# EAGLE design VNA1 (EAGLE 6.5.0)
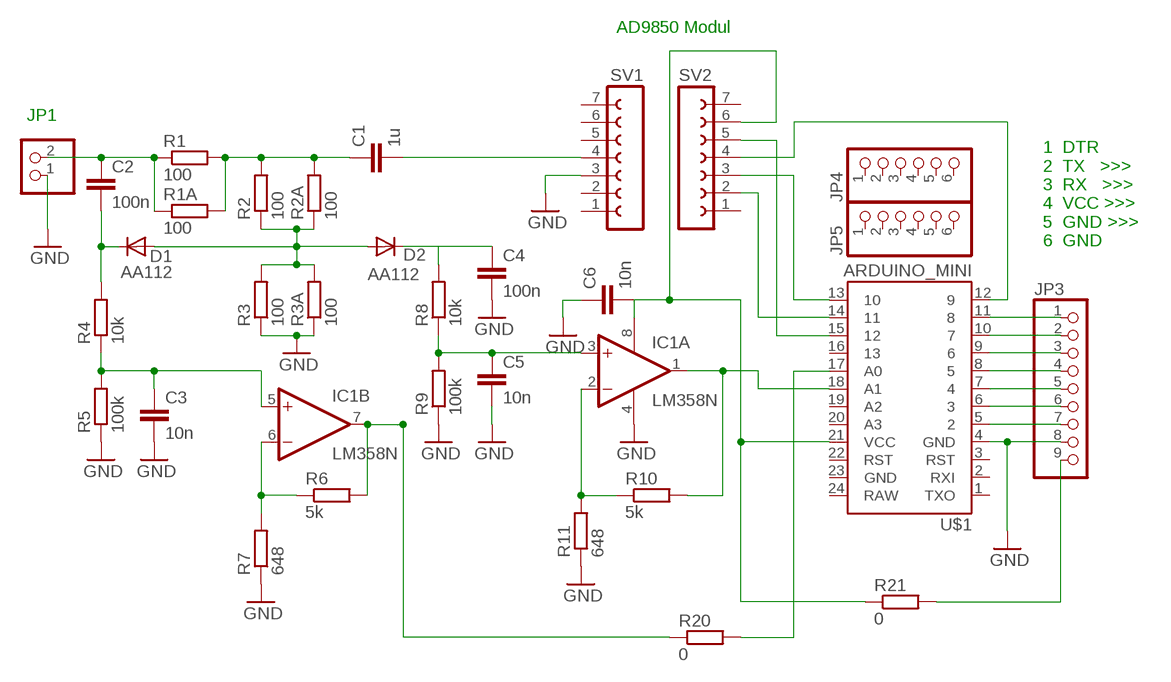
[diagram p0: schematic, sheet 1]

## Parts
C1  1u  C-EU025-040X050  [C025-040X050]
C2  100n  C-EU050-025X075  [C050-025X075]
C3  10n  C-EU050-025X075  [C050-025X075]
C4  100n  C-EU050-025X075  [C050-025X075]
C5  10n  C-EU050-025X075  [C050-025X075]
C6  10n  C-EU050-025X075  [C050-025X075]
D1  AA112  [DO07]
D2  AA112  [DO07]
IC1  LM358N  [DIL08]
JP1  PINHD-1X2  [1X02]
JP3  PINHD-1X9  [1X09]
JP4  PINHD-1X6  [1X06]
JP5  PINHD-1X6  [1X06]
R1  100  R-EU_0207/7  [0207/7]
R1A  100  R-EU_0207/7  [0207/7]
R2  100  R-EU_0207/7  [0207/7]
R2A  100  R-EU_0207/7  [0207/7]
R3  100  R-EU_0207/7  [0207/7]
R3A  100  R-EU_0207/7  [0207/7]
R4  10k  R-EU_0207/7  [0207/7]
R5  100k  R-EU_0207/7  [0207/7]
R6  5k  R-EU_0207/7  [0207/7]
R7  648  R-EU_0207/7  [0207/7]
R8  10k  R-EU_0207/7  [0207/7]
R9  100k  R-EU_0207/7  [0207/7]
R10  5k  R-EU_0207/7  [0207/7]
R11  648  R-EU_0207/7  [0207/7]
R20  0  R-EU_0207/7  [0207/7]
R21  0  R-EU_0207/7  [0207/7]
SV1  FE07-1  [FE07]
SV2  FE07-1  [FE07]
U$1  ARDUINO_MINI  [ARDUINO_MINI]

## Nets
GND: C3.2 C4.2 C5.2 C6.1 IC1.4(P:V-) JP1.1 JP3.8 R3.1 R3A.1 R5.1 R7.1 R9.1 R11.1 SV1.3 U$1.4(GND)
N$1: C3.1 IC1.5(B:+IN) R4.1 R5.2
N$2: C2.1 JP1.2 R1.1 R1A.1
N$3: C1.1 R1.2 R1A.2 R2.2 R2A.2
N$4: C2.2 D1.C R4.2
N$5: D1.A D2.A R2.1 R2A.1 R3.2 R3A.2
N$6: IC1.6(B:-IN) R6.1 R7.2
N$7: C4.1 D2.C R8.2
N$8: IC1.7(B:OUT) R6.2 R20.1
N$9: C5.1 IC1.3(A:+IN) R8.1 R9.2
N$10: IC1.2(A:-IN) R10.1 R11.2
N$12: C1.2 SV1.4
N$14: C6.2 IC1.8(P:V+) R21.1 SV2.6 U$1.21(VCC)
N$15: SV2.5 U$1.15
N$16: SV2.3 U$1.13
N$17: SV2.4 U$1.12
N$18: SV2.2 U$1.14
N$19: R20.2 U$1.17(A0)
N$20: JP3.9 R21.2
N$21: JP3.1 U$1.11
N$22: JP3.2 U$1.10
N$23: JP3.3 U$1.9
N$24: JP3.4 U$1.8
N$25: JP3.5 U$1.7
N$26: JP3.6 U$1.6
N$27: JP3.7 U$1.5
N$28: IC1.1(A:OUT) R10.2 U$1.18(A1)
Unconnected: JP4.1 JP4.2 JP4.3 JP4.4 JP4.5 JP4.6 JP5.1 JP5.2 JP5.3 JP5.4 JP5.5 JP5.6 SV1.1 SV1.2 SV1.5 SV1.6 SV1.7 SV2.1 SV2.7 U$1.1(TXO) U$1.2(RXI) U$1.3(RST) U$1.16 U$1.19(A2) U$1.20(A3) U$1.22(RST) U$1.23(GND) U$1.24(RAW)

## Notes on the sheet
- AD9850 Modul
- 1  DTR
  2  TX   >>>
  3  RX   >>>
  4  VCC >>>
  5  GND >>>
  6  GND

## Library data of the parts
C1-C6 = resistor:C-EU: CAPACITOR, European symbol
D1 D2 = diode:AA112: DIODE
IC1 = linear:LM358: OP AMP also LM158; LM258; LM2904 Source: http://cache.national.com/ds/LM/LM158.pdf
JP1 = pinhead:PINHD-1X2: PIN HEADER
JP3 = pinhead:PINHD-1X9: PIN HEADER
JP4 JP5 = pinhead:PINHD-1X6: PIN HEADER
R1 R1A R2 R2A R3 R3A R4-R11 R20 R21 = resistor:R-EU_: RESISTOR, European symbol
SV1 SV2 = con-lsta:FE07-1: FEMALE HEADER; OC_FARNELL: unknown; OC_NEWARK: unknown
U$1 = sparkfun_boards:ARDUINO_MINI: Arduino Pro Mini footprint

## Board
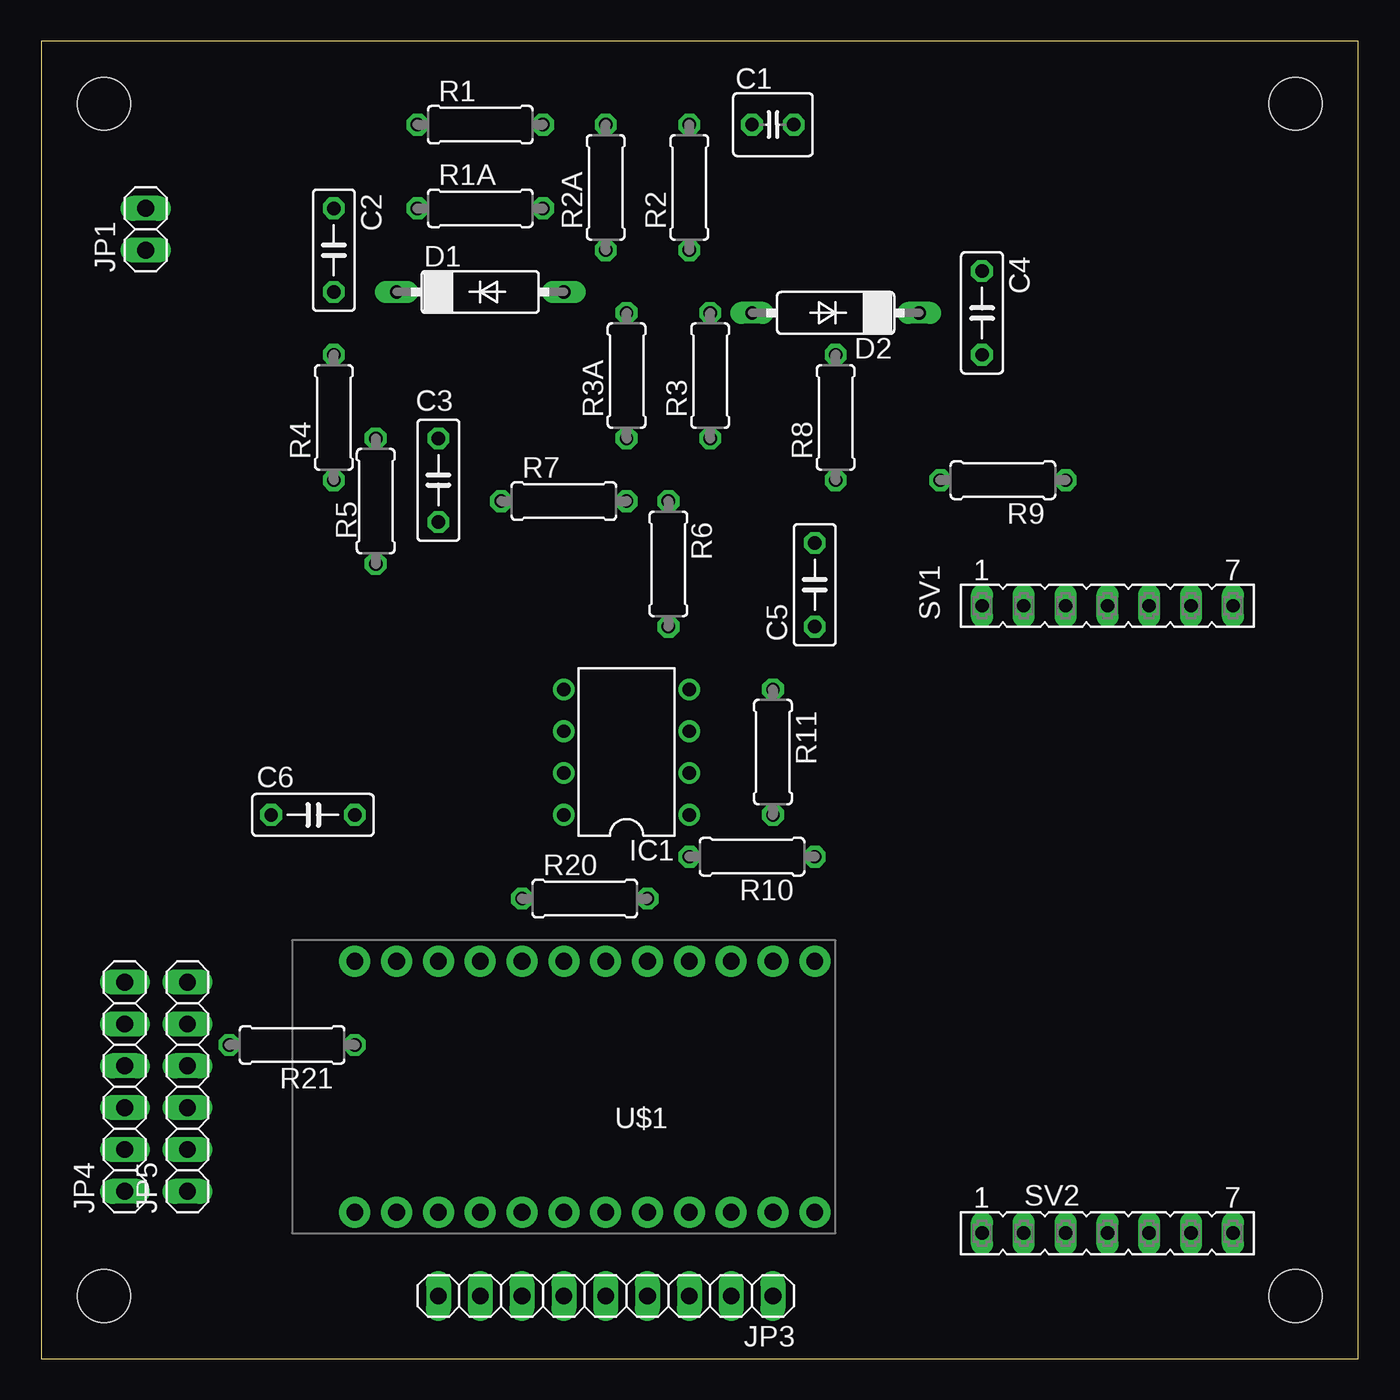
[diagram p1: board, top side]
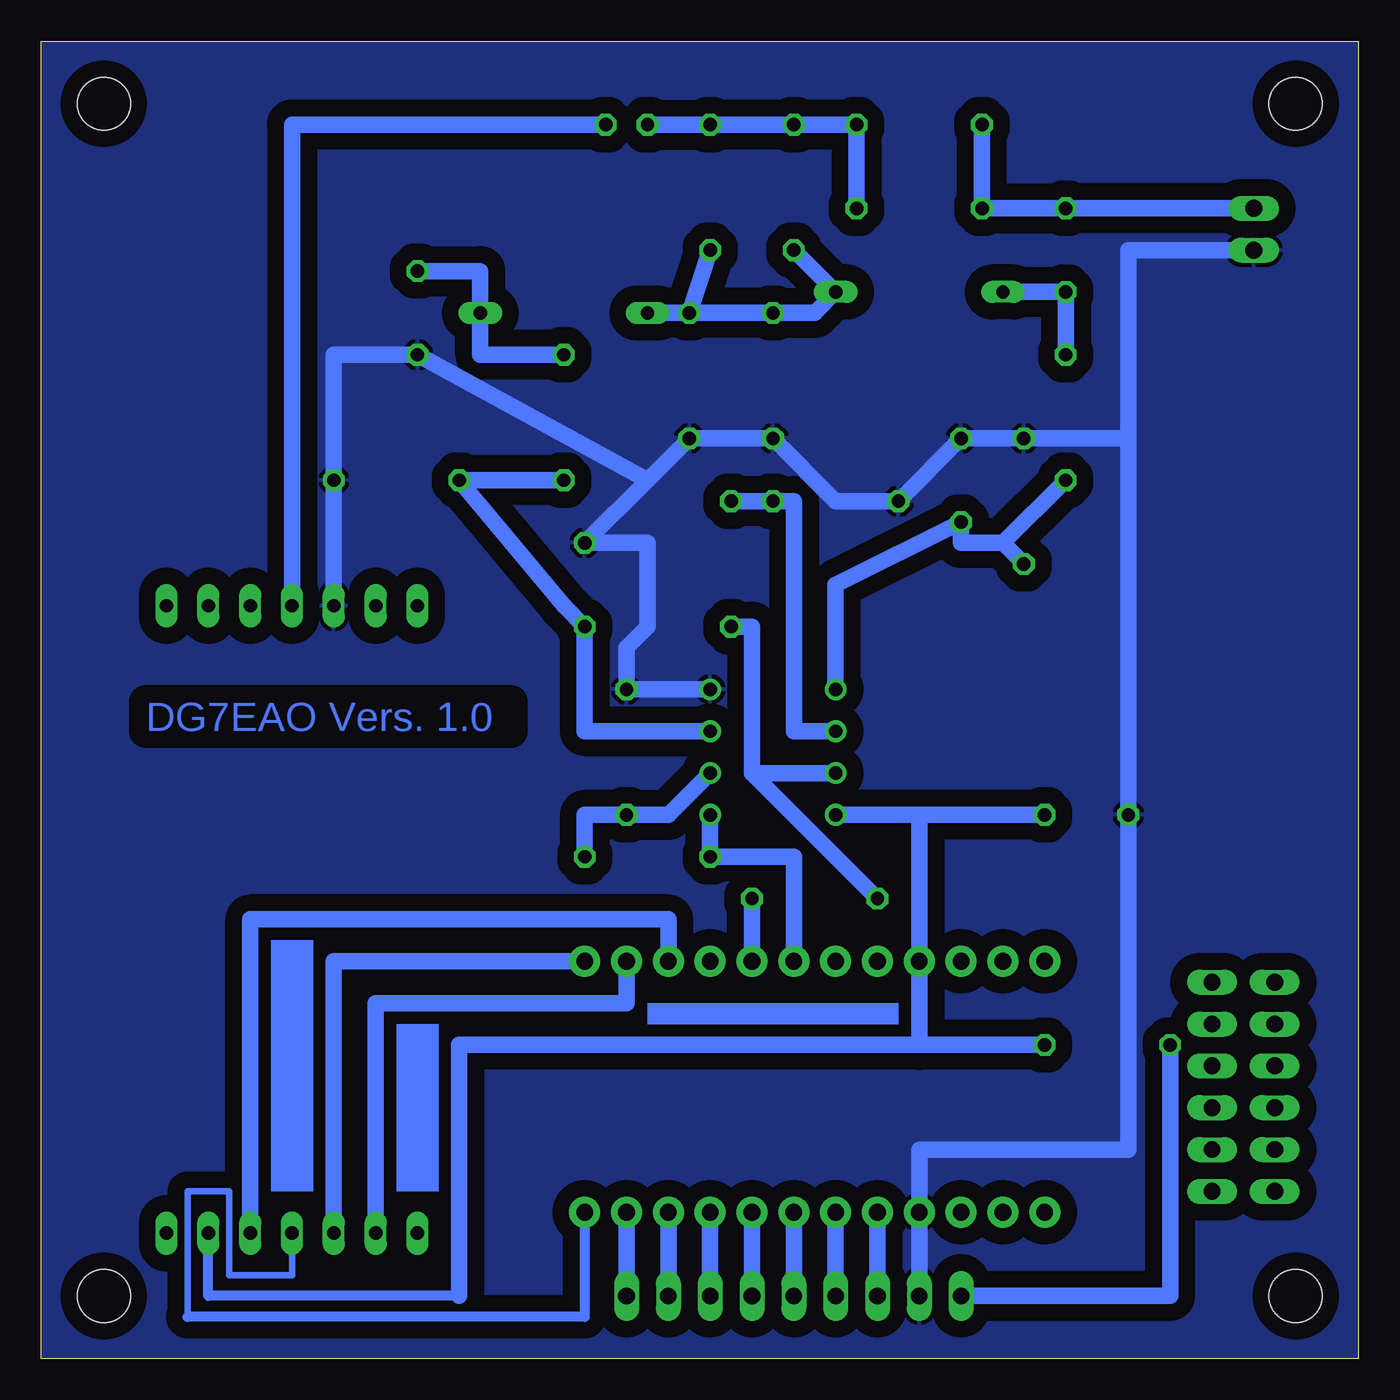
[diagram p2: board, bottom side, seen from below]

Size 80.01 x 80 mm. Coordinates in mm from the lower left corner, seen from the top.
Outline: 0,0 80.01,0 80,80 0,80 0,0
Copper layers (1*16): Top 0.035mm / dielectric 1.5mm / Bottom 0.035mm
Design rules "default *": minimum track width 10mil, minimum drill 24mil, track to track 8mil, track to pad 8mil, pad to pad 8mil, via to via 8mil, smd to smd 8mil, copper to edge 0mil, drill to drill 8mil, minimum pad ring 10mil, minimum via ring 8mil, stop-mask expansion 4mil, vias tented up to drill 0mil, thermal gap 10mil
Holes 3.2 mm at 3.81,76.2 3.81,3.81 76.2,76.2 76.2,3.81

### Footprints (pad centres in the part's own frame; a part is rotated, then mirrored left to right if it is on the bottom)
C025-040X050 = drill 0.813 octagon: 1 -1.27,0; 2 1.27,0
C050-025X075 = drill 0.813 octagon: 1 -2.54,0; 2 2.54,0
DO07 = drill 0.813 long: A 5.08,0; C -5.08,0
DIL08 = drill 0.813 pad 1.27: 1 -3.81,-3.81; 2 -1.27,-3.81; 3 1.27,-3.81; 4 3.81,-3.81; 5 3.81,3.81; 6 1.27,3.81; 7 -1.27,3.81; 8 -3.81,3.81
1X02 = drill 1.016 long: 1 -1.27,0; 2 1.27,0
1X09 = drill 1.016 long: 1 -10.16,0; 2 -7.62,0; 3 -5.08,0; 4 -2.54,0; 5 0,0; 6 2.54,0; 7 5.08,0; 8 7.62,0; 9 10.16,0
1X06 = drill 1.016 long: 1 -6.35,0; 2 -3.81,0; 3 -1.27,0; 4 1.27,0; 5 3.81,0; 6 6.35,0
0207/7 = drill 0.813 octagon: 1 -3.81,0; 2 3.81,0
FE07 = drill 0.813 long: 1 -7.62,0; 2 -5.08,0; 3 -2.54,0; 4 0,0; 5 2.54,0; 6 5.08,0; 7 7.62,0
ARDUINO_MINI = drill 1.016 pad 1.88: 1 -7.62,12.7; 2 -7.62,10.16; 3 -7.62,7.62; 4 -7.62,5.08; 5 -7.62,2.54; 6 -7.62,0; 7 -7.62,-2.54; 8 -7.62,-5.08; 9 -7.62,-7.62; 10 -7.62,-10.16; 11 -7.62,-12.7; 12 -7.62,-15.24; 13 7.62,-15.24; 14 7.62,-12.7; 15 7.62,-10.16; 16 7.62,-7.62; 17 7.62,-5.08; 18 7.62,-2.54; 19 7.62,0; 20 7.62,2.54; 21 7.62,5.08; 22 7.62,7.62; 23 7.62,10.16; 24 7.62,12.7

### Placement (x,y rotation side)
C1  44.45,74.93 0 top
C2  17.78,67.31 270 top
C3  24.13,53.34 90 top
C4  57.15,63.5 270 top
C5  46.99,46.99 90 top
C6  16.51,33.02 0 top
D1  26.67,64.77 0 top
D2  48.26,63.5 180 top
IC1  35.56,36.83 90 top
JP1  6.35,68.58 90 top
JP3  34.29,3.81 180 top
JP4  5.08,16.51 90 top
JP5  8.89,16.51 90 top
R1  26.67,74.93 0 top
R1A  26.67,69.85 0 top
R2  39.37,71.12 90 top
R2A  34.29,71.12 90 top
R3  40.64,59.69 90 top
R3A  35.56,59.69 90 top
R4  17.78,57.15 90 top
R5  20.32,52.07 270 top
R6  38.1,48.26 270 top
R7  31.75,52.07 0 top
R8  48.26,57.15 90 top
R9  58.42,53.34 180 top
R10  43.18,30.48 180 top
R11  44.45,36.83 270 top
R20  33.02,27.94 0 top
R21  15.24,19.05 180 top
SV1  64.77,45.72 0 top
SV2  64.77,7.62 0 top
U$1  31.75,16.51 90 top

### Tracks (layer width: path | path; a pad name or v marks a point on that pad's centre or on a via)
GND
  Bottom 1.016: IC1.4 R11.1 44.45,43.18 43.18,44.45 43.18,49.53 C5.2 43.18,53.34 | 43.18,53.34 R3.1 R3A.1 31.75,52.07 R7.1 C3.2 R5.1 13.97,55.88 | 43.18,53.34 C4.2 62.23,60.96 R9.1 SV1.3 | JP3.8 U$1.4 26.67,12.7 13.97,12.7 C6.1 13.97,55.88 | JP1.1 13.97,67.31 13.97,55.88
  pour Bottom (isolate 1.016): 0,80.01 80.01,80.01 80.01,0 0,0
N$1
  Bottom 1.016: 21.59,49.53 24.13,49.53 C3.1 31.75,46.99 IC1.5 | 21.59,49.53 R5.2 | 21.59,49.53 R4.1
N$2
  Bottom 1.016: R1.1 R1A.1 C2.1 JP1.2
N$3
  Bottom 1.016: R1A.2 R1.2 R2A.2 R2.2 C1.1
N$4
  Bottom 1.016: D1.C C2.2 R4.2
N$5
  Bottom 1.016: R2.1 R3.2 | R2A.1 D1.A 33.02,63.5 R3A.2 R3.2 | R3.2 D2.A
N$6
  Bottom 1.016: IC1.6 34.29,38.1 34.29,52.07 R7.2 R6.1
N$7
  Bottom 1.016: C4.1 53.34,66.04 D2.C 53.34,60.96 R8.2
N$8
  Bottom 1.016: R6.2 36.83,44.45 36.83,35.56 | 36.83,35.56 IC1.7 | 36.83,35.56 R20.1
N$9
  Bottom 1.016: R8.1 R9.2 48.26,45.72 C5.1 46.99,38.1 IC1.3
N$10
  Bottom 1.016: R10.1 46.99,33.02 R11.2 41.91,33.02 IC1.2
N$12
  Bottom 1.016: SV1.4 64.77,74.93 C1.2
N$14
  Bottom 0.61: 54.61,3.81 69.85,3.81 SV2.6
  Bottom 1.016: C6.2 26.67,33.02 | 26.67,33.02 IC1.8 | 26.67,33.02 U$1.21 26.67,19.05 | 26.67,19.05 54.61,19.05 54.61,3.81 | R21.1 26.67,19.05
N$15
  Bottom 1.016: U$1.15 41.91,26.67 67.31,26.67 SV2.5
N$16
  Bottom 1.016: U$1.13 62.23,24.13 SV2.3
N$17
  Bottom 0.406: 71.12,2.54 71.12,10.16 68.58,10.16 68.58,5.08 64.77,5.08 SV2.4
  Bottom 0.61: U$1.12 46.99,2.54 71.12,2.54
N$18
  Bottom 1.016: U$1.14 44.45,21.59 59.69,21.59 SV2.2
N$19
  Bottom 1.016: U$1.17 R20.2
N$20
  Bottom 1.016: JP3.9 11.43,3.81 R21.2
N$21
  Bottom 1.016: U$1.11 JP3.1
N$22
  Bottom 1.016: U$1.10 JP3.2
N$23
  Bottom 1.016: U$1.9 JP3.3
N$24
  Bottom 1.016: U$1.8 JP3.4
N$25
  Bottom 1.016: U$1.7 JP3.5
N$26
  Bottom 1.016: U$1.6 JP3.6
N$27
  Bottom 1.016: U$1.5 JP3.7
N$28
  Bottom 1.016: U$1.18 34.29,30.48 R10.2 IC1.1
(copper drawn outside any net)
  shapes: Bottom area x3

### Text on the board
Bottom: DG7EAO Vers. 1.0

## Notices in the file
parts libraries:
sparkfun_boards: Licensing: Creative Commons ShareAlike 4.0 International - https://creativecommons.org/licenses/by-sa/4.0
